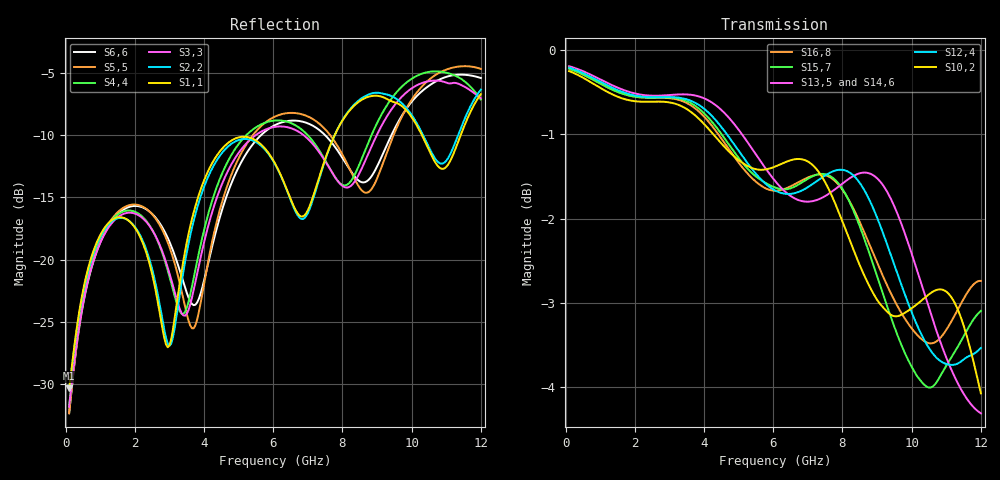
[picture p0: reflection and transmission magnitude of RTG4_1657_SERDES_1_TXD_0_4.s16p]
! RTG4 1657 S-parameter file
! Microsemi Corporation (c) 2019
!Initial ver: Jul 30, 2019
! Port::PIN_NAME::NET_NAME::S-parameter ports::PORT SIDE
! Port1:--:SERDES_1_TXD0_N_DIE::1::DIE
! Port2:--:SERDES_1_TXD0_P_DIE::2::DIE
! Port3:AT9:SERDES_1_TXD0_N_BGA::3::BGA
! Port4:AU9:SERDES_1_TXD0_P_BGA::4::BGA
! Port5:--:SERDES_1_TXD1_N_DIE::5::DIE
! Port6:--:SERDES_1_TXD1_P_DIE::6::DIE
! Port7:AT11:SERDES_1_TXD1_N_BGA::7::BGA
! Port8:AU11:SERDES_1_TXD1_P_BGA::8::BGA
! Port9:--:SERDES_1_TXD2_N_DIE::9::DIE
! Port10:--:SERDES_1_TXD2_P_DIE::10::DIE
! Port11:AT13:SERDES_1_TXD2_N_BGA::11::BGA
! Port12:AU13:SERDES_1_TXD2_P_BGA::12::BGA
! Port13:--:SERDES_1_TXD3_N_DIE::13::DIE
! Port14:--:SERDES_1_TXD3_P_DIE::14::DIE
! Port15:AV14:SERDES_1_TXD3_N_BGA::15::BGA
! Port16:AW14:SERDES_1_TXD3_P_BGA::16::BGA
!TouchstoneFormatFlag = 1
! GNDNET
! NETSLIST
! User Comments:
! Touchstone file exported from HFSS 2018.2.0
!  File:  L:/LSI/Simulation/MASUMIZU/MicroSemi/190627_KD-YB5197_Spara/End/YBD197_150320_NETCHANGE_SERDES_1_TXD1.aedt
!  Generated:  9:25:36  7 09, 2019
!  Design:  HFSSModel1
!  Project:  YBD197_150320_NETCHANGE_SERDES_1_TXD1
!  Setup:  Setup1
!  Solution:  Sweep
! Terminal data exported
! Port[1] = SERDES_1_TXD0_N_DIE
! Port[2] = SERDES_1_TXD0_P_DIE
! Port[3] = SERDES_1_TXD1_N_DIE
! Port[4] = SERDES_1_TXD1_P_DIE
! Port[5] = SERDES_1_TXD2_N_DIE
! Port[6] = SERDES_1_TXD2_P_DIE
! Port[7] = SERDES_1_TXD3_N_DIE
! Port[8] = SERDES_1_TXD3_P_DIE
! Port[9] = SERDES_1_TXD0_N_BGA
! Port[10] = SERDES_1_TXD0_P_BGA
! Port[11] = SERDES_1_TXD1_N_BGA
! Port[12] = SERDES_1_TXD1_P_BGA
! Port[13] = SERDES_1_TXD2_N_BGA
! Port[14] = SERDES_1_TXD2_P_BGA
! Port[15] = SERDES_1_TXD3_N_BGA
! Port[16] = SERDES_1_TXD3_P_BGA
# GHZ S DB R 50.000000
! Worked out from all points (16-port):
!   239 points, 100 MHz to 12 GHz, reference 50 ohm
!   strongest paths, dB at 100 MHz, 3.05 GHz, 6.05 GHz, 9.05 GHz, 12 GHz:
!     S10,2: -0.2, -0.6, -1.4, -3.0, -4.1
!     S12,4: -0.2, -0.6, -1.7, -2.0, -3.5
!     S13,5: -0.2, -0.5, -1.6, -1.5, -4.3
!     S14,6: -0.2, -0.5, -1.5, -1.6, -4.3
!     S15,7: -0.2, -0.6, -1.6, -2.7, -3.1
!     S16,8: -0.2, -0.6, -1.7, -2.6, -2.7
!   lowest |S11| = -30.3 dB at 100 MHz (marker M1), VSWR 1.06, Z = 52.6 - j1.67 ohm
!   |S11| at or under -10 dB: start of sweep to 7.774 GHz; 10.3 GHz to 11.42 GHz (1.12 GHz wide, 10.3 % of centre)
